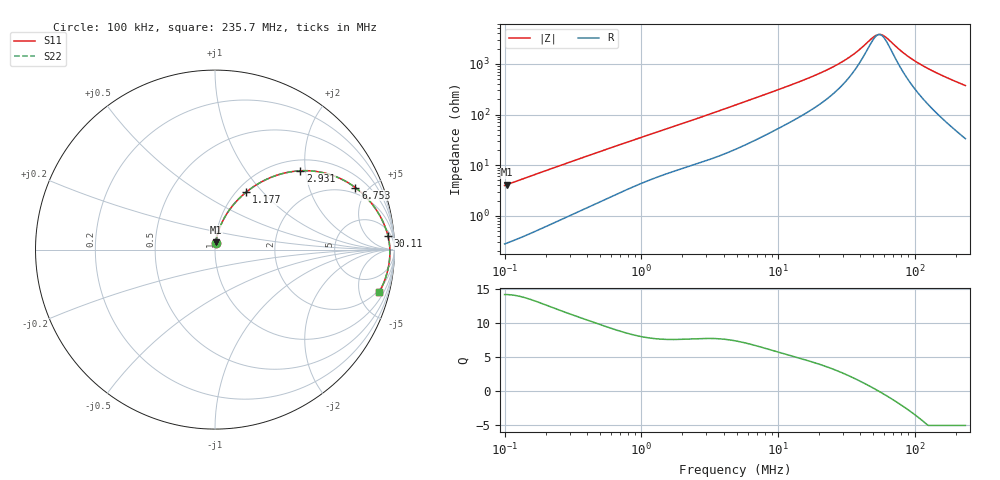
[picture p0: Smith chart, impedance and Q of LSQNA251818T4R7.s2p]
! LSQNA251818T4R7  S-PARAMETER MODEL  ( General Type )
! Model Generated by TAIYO YUDEN Corporation (http://www.ty-top.com)
! Version 2.0
! TAIYO YUDEN Control No. 100810NF25SB-FKC
! Copyright(c) 2007 TAIYO YUDEN CO.,LTD. All Rights Reserved.
! Product Description (link to TY-COMPAS)
! https://ds.yuden.co.jp/TYCOMPAS/or/detail?pn=LSQNA251818T4R7M&u=M
! Products Name : Inductors
! Characteristics :
!  Inductance : 4.7 uH , SRF(min) : 46 MHz , DC Resistance(max) : 0.169 Ohm
!  Rated Current : Saturation :340 mA , Temp Rise : 1100 mA (40 degC)
!  Case Size : 2.5 x 1.8 / 0.098 x 0.071 [mm/inch] , Thickness : 1.8 / 0.071 [mm/inch]
!  (Conditions: Temperature = 25 degC , DC Bias Current/Voltage = 0A / 0V)
! External Node Assignments :
!  1  o---GGG---o  2
! GND o---------o GND
! Frequency Range : 0.1MHz  -  235.669543MHz  [ 402 STEP ]
# MHz S RI R 50
! Freq[MHz].  S11 Real  S11 Imag  S21 Real  S21 Imag  S12 Real  S12 Imag  S22 Real  S22 Imag
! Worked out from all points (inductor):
!   401 points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, 100 kHz to 235.7 MHz, reference 50 ohm
!   read as one part in series: L = 6.29 uH near 104 kHz
!   highest Q = 14.2 at 104 kHz (marker M1), where L = 6.32 uH
!   self-resonance near 55.09 MHz
!   S11 on the Smith chart (normalised r, x): 100 kHz: 1.01, +0.08; 1.177 MHz: 1.10, +0.81; 2.931 MHz: 1.24, +1.88; 6.753 MHz: 1.61, +4.15; 30.11 MHz: 9, +21; 235.7 MHz: 1.67, -7.42
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0.1  0.00435 0.0394  0.9956 -0.0394  0.9956 -0.0394  0.00435 0.0394
0.103959  0.00458 0.041  0.9954 -0.041  0.9954 -0.041  0.00458 0.041
0.367165  0.0309 0.1327  0.9691 -0.1327  0.9691 -0.1327  0.0309 0.1327
0.683353  0.0806 0.2218  0.9194 -0.2218  0.9194 -0.2218  0.0806 0.2218
1.17681  0.1732 0.3197  0.8268 -0.3197  0.8268 -0.3197  0.1732 0.3197
1.348099  0.206 0.3446  0.794 -0.3446  0.794 -0.3446  0.206 0.3446
1.949423  0.3175 0.4046  0.6825 -0.4046  0.6825 -0.4046  0.3175 0.4046
2.930569  0.4753 0.4392  0.5247 -0.4392  0.5247 -0.4392  0.4753 0.4392
4.854581  0.6782 0.4047  0.3218 -0.4047  0.3218 -0.4047  0.6782 0.4047
6.752656  0.7828 0.345  0.2172 -0.345  0.2172 -0.345  0.7828 0.345
10.55315  0.8762 0.2524  0.1238 -0.2524  0.1238 -0.2524  0.8762 0.2524
17.8243  0.9354 0.156  0.0646 -0.156  0.0646 -0.156  0.9354 0.156
30.10531  0.9635 0.0773  0.0365 -0.0773  0.0365 -0.0773  0.9635 0.0773
37.27189  0.9694 0.0491  0.0306 -0.0491  0.0306 -0.0491  0.9694 0.0491
48.91162  0.9736 0.0148  0.0264 -0.0148  0.0264 -0.0148  0.9736 0.0148
52.86096  0.9742 0.00513  0.0258 -0.00513  0.0258 -0.00513  0.9742 0.00513
58.24905  0.9746 -0.00696  0.0254 0.00696  0.0254 0.00696  0.9746 -0.00696
65.44454  0.9746 -0.0216  0.0254 0.0216  0.0254 0.0216  0.9746 -0.0216
84.23125  0.9726 -0.0547  0.0274 0.0547  0.0274 0.0547  0.9726 -0.0547
108.4109  0.9675 -0.0909  0.0325 0.0909  0.0325 0.0909  0.9675 -0.0909
156.768  0.9518 -0.1531  0.0482 0.1531  0.0482 0.1531  0.9518 -0.1531
235.6695  0.9143 -0.2386  0.0857 0.2386  0.0857 0.2386  0.9143 -0.2386
